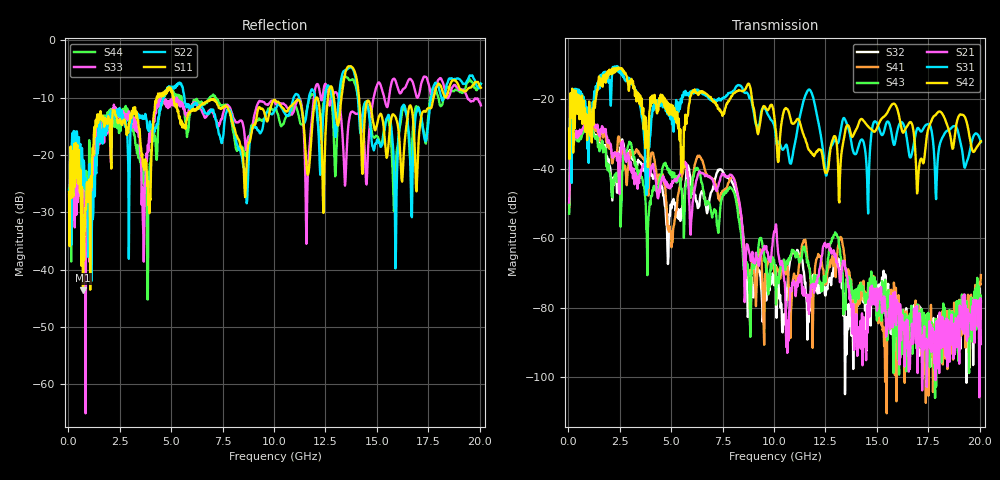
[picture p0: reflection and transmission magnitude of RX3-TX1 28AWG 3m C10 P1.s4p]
! FILE: O:\PROJECTS\SI-2007-05-003 3m Eyemax Qual\XT\FD\RX3-TX1 28AWG 3m C10 P1.s4p
# MHZ S RI R 50.00
! FREQ  S11  S12  S13  S14
!  S21  S22  S23  S24
!  S31  S32  S33  S34
!  S41  S42  S43  S44
!  REAL  IMAG  REAL  IMAG  REAL  IMAG  REAL  IMAG
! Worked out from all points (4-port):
!   801 points, 50 MHz to 20.05 GHz, reference 50 ohm
!   strongest paths, dB at 50 MHz, 5.05 GHz, 10.05 GHz, 15.05 GHz, 20.05 GHz:
!     S42: -28.5, -24.5, -26.7, -27.6, -32.1
!     S31: -29.0, -27.3, -28.7, -27.5, -32.4
!     S21: -49.8, -44.2, -58.1, -77.8, -90.5
!     S43: -53.0, -42.5, -68.0, -77.0, -78.4
!     S41: -52.4, -61.2, -69.4, -76.7, -70.6
!     S32: -50.2, -49.4, -68.7, -75.7, -78.2
!   lowest |S11| = -43.6 dB at 725 MHz (marker M1), VSWR 1.01, Z = 50.1 + j0.652 ohm
!   |S11| at or under -10 dB: start of sweep to 4.299 GHz; 5.13 GHz to 12.05 GHz (6.917 GHz wide, 80.5 % of centre); 14.13 GHz to 17.75 GHz (3.624 GHz wide, 22.7 % of centre)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
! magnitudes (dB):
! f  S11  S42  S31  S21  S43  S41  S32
! 50 MHz  -26.4  -28.5  -29.0  -49.8  -53.0  -52.4  -50.2
! 725 MHz  -43.6  -23.3  -25.6  -28.3  -29.7  -28.6  -29.4
! 4.85 GHz  -8.8  -21.0  -21.2  -44.5  -40.0  -57.3  -67.5
! 7.475 GHz  -11.8  -24.2  -19.8  -41.4  -48.5  -46.7  -40.4
! 8.8 GHz  -17.8  -15.7  -19.6  -64.3  -73.1  -69.6  -76.3
! 12.53 GHz  -14.5  -41.2  -42.0  -62.1  -70.8  -73.1  -75.5
! 20.05 GHz  -8.3  -32.1  -32.4  -90.5  -78.4  -70.6  -78.2
